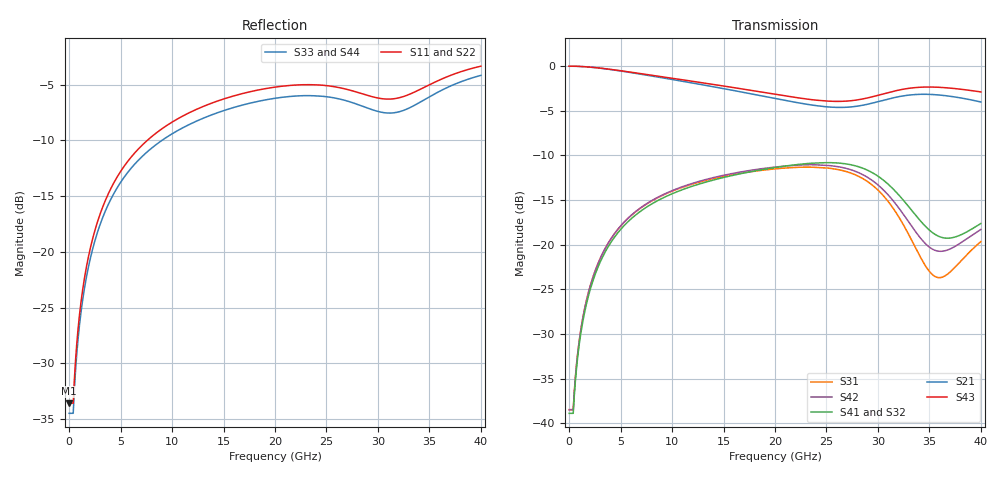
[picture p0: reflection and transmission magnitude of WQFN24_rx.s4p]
! Created Fri Aug 22 08:00:57 2014
# hz S db R 50
! 4 Port Network Data from SP1.SP block
! freq  dbS11  angS11  dbS12  angS12  dbS13  angS13  dbS14  angS14
!  dbS21  angS21  dbS22  angS22  dbS23  angS23  dbS24  angS24
!  dbS31  angS31  dbS32  angS32  dbS33  angS33  dbS34  angS34
!  dbS41  angS41  dbS42  angS42  dbS43  angS43  dbS44  angS44
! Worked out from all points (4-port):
!   4001 points, 1 MHz to 40 GHz, reference 50 ohm
!   strongest paths, dB at 1 MHz, 10 GHz, 20 GHz, 30 GHz, 40 GHz:
!     S43: 0.0, -1.4, -3.2, -3.3, -2.9
!     S21: 0.0, -1.5, -3.6, -4.0, -4.0
!     S41: -38.9, -14.3, -11.4, -12.3, -17.6
!     S32: -38.9, -14.3, -11.4, -12.3, -17.4
!     S42: -38.5, -14.0, -11.3, -13.3, -18.3
!     S31: -38.5, -14.0, -11.5, -13.9, -19.7
!   lowest |S11| = -33.6 dB at 1 MHz (marker M1), VSWR 1.04, Z = 50.1 + j2.1 ohm
!   |S11| at or under -10 dB: start of sweep to 7.585 GHz
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1000000  -33.57 85.8  -0.01 -1.6  -38.48 85.7  -38.89 -94.3
         -0.01 -1.6  -33.57 86.1  -38.90 -94.3  -38.50 86.0
         -38.48 85.7  -38.90 -94.3  -34.49 85.7  -0.01 -1.4
         -38.89 -94.3  -38.50 86.0  -0.01 -1.4  -34.49 86.1
1.521e9  -22.19 79.6  -0.07 -5.8  -27.10 76.3  -27.50 -103.6
         -0.07 -5.8  -22.19 80.9  -27.50 -103.6  -27.10 77.6
         -27.10 76.3  -27.50 -103.6  -23.11 79.4  -0.07 -5.4
         -27.50 -103.6  -27.10 77.6  -0.07 -5.4  -23.11 80.8
3.111e9  -16.35 70.8  -0.25 -11.5  -21.33 63.6  -21.72 -116.1
         -0.25 -11.5  -16.35 73.4  -21.72 -116.2  -21.32 66.2
         -21.33 63.6  -21.72 -116.2  -17.29 70.4  -0.24 -10.7
         -21.72 -116.1  -21.32 66.2  -0.24 -10.7  -17.29 73.3
9.951e9  -8.38 42.0  -1.49 -30.9  -14.03 21.4  -14.33 -157.5
         -1.49 -30.9  -8.39 50.2  -14.33 -157.9  -13.98 29.7
         -14.03 21.4  -14.33 -157.9  -9.43 41.8  -1.35 -28.2
         -14.33 -157.5  -13.98 29.7  -1.35 -28.2  -9.44 51.0
2.5811e10  -5.18 -4.8  -4.62 -51.5  -11.53 -60.5  -10.83 125.3
           -4.62 -51.5  -5.18 16.9  -10.84 124.5  -11.21 -37.7
           -11.53 -60.5  -10.84 124.5  -6.19 -4.6  -3.95 -47.7
           -10.83 125.3  -11.21 -37.7  -3.95 -47.7  -6.24 19.5
3.5581e10  -4.74 -4.4  -3.20 -67.4  -23.59 -85.0  -18.87 91.4
           -3.20 -67.4  -4.75 24.1  -18.66 91.7  -20.65 -55.0
           -23.59 -85.0  -18.66 91.7  -5.78 -0.8  -2.36 -63.4
           -18.87 91.4  -20.65 -55.0  -2.36 -63.4  -5.85 31.7
4e10  -3.33 -14.7  -4.02 -79.3  -19.66 -57.8  -17.63 112.0
      -4.02 -79.3  -3.45 18.2  -17.39 110.7  -18.30 -32.9
      -19.66 -57.8  -17.39 110.7  -4.16 -10.2  -2.89 -75.2
      -17.63 112.0  -18.30 -32.9  -2.89 -75.2  -4.28 26.7
